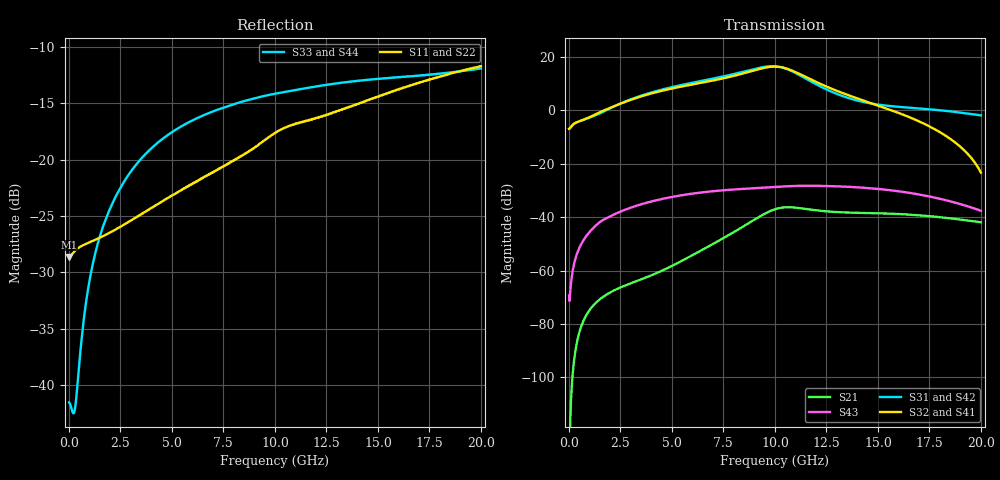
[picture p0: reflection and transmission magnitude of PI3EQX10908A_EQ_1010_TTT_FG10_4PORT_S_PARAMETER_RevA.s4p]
! NPort=4 DATA=2000 NOISE=0 GROUPDELAY=0 COMPLEX_DATAFORMAT=POLAR
! NumOfBlock=1 NumOfParam=0
! .MODEL Smodel S TSTONEFILE=PI3EQX10908A_EQ_1010_TTT_FG10_4PORT_S_PARAMETER_RevA.s4p TYPE=S
!  -- The above .MODEL line can be used for the S element in the netlist.
! The s parameter is extracted from the linear redriver, it is not bi-directional; only s(4,1)s(4,2) and s(3,1)s(3,2)
! should be the insertion loss
!Port definition:
!Port1 = input+
!Port2 = input-
!Port3 = output+
!Port4 = output-
# Hz S MA R  50
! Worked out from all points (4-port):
!   2000 points, 10 MHz to 20 GHz, reference 50 ohm
!   strongest paths, dB at 10 MHz, 5.01 GHz, 10.01 GHz, 15.01 GHz, 20 GHz:
!     S32: -6.9, 8.2, 16.3, 1.8, -23.3
!     S41: -6.9, 8.2, 16.3, 1.8, -23.3
!     S31: -6.9, 8.7, 16.5, 2.1, -1.9
!     S42: -6.9, 8.7, 16.5, 2.1, -1.9
!     S43: -69.4, -32.4, -28.7, -29.5, -37.6
!     S21: -127.2, -58.2, -37.0, -38.6, -41.9
!   lowest |S11| = -28.6 dB at 10 MHz (marker M1), VSWR 1.08, Z = 46.4 - j0.024 ohm
!   |S11| at or under -10 dB: start of sweep to end of sweep
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1e7  0.03701 -179.6  4.341e-07 14.5  0 0.0  0 0.0
     4.341e-07 14.5  0.03701 -179.6  0 0.0  0 0.0
     0.4507 1.1  0.4507 -178.9  0.008374 26.0  0.00034 -27.1
     0.4507 -178.9  0.4507 1.1  0.00034 -27.1  0.008374 26.0
6.85e9  0.08649 -119.6  0.002926 133.9  4.484e-07 62.9  2.294e-07 136.3
        0.002926 134.0  0.08652 -119.6  2.294e-07 136.3  4.484e-07 62.8
        3.821 -51.5  3.517 122.0  0.1617 10.9  0.03013 15.2
        3.518 122.0  3.821 -51.5  0.03013 15.2  0.1617 10.9
9.18e9  0.116 -111.6  0.009814 111.4  2.651e-06 18.1  1.658e-06 115.9
        0.009818 111.4  0.116 -111.6  1.659e-06 115.9  2.651e-06 18.1
        6.164 -111.5  5.847 63.0  0.1889 -7.1  0.035 -8.7
        5.847 63.0  6.165 -111.5  0.035 -8.7  0.1889 -7.1
1.035e10  0.1369 -112.0  0.01505 73.8  4.316e-06 -16.1  4.594e-06 81.4
          0.01506 73.8  0.137 -112.0  4.596e-06 81.5  4.316e-06 -16.2
          6.34 -163.9  6.344 9.6  0.1987 -14.9  0.03735 -20.6
          6.344 9.6  6.341 -163.9  0.03735 -20.6  0.1987 -14.9
1.143e10  0.1478 -113.4  0.01434 42.4  5.025e-06 -26.0  7.712e-06 44.7
          0.01434 42.4  0.1479 -113.4  7.715e-06 44.7  5.024e-06 -26.1
          4.059 155.2  4.338 -34.8  0.207 -21.1  0.03852 -33.7
          4.337 -34.7  4.059 155.2  0.03852 -33.7  0.207 -21.1
1.361e10  0.1718 -111.8  0.01214 14.6  1.366e-05 -36.4  1.654e-05 -5.1
          0.01213 14.7  0.1719 -111.8  1.655e-05 -5.1  1.365e-05 -36.5
          1.679 125.7  1.89 -82.4  0.2216 -32.5  0.03681 -60.1
          1.889 -82.4  1.679 125.7  0.03681 -60.1  0.2216 -32.5
2e10  0.2599 -114.7  0.008018 -40.2  8.927e-05 -147.8  7.211e-05 -138.7
      0.008014 -39.9  0.2601 -114.7  7.212e-05 -138.7  8.925e-05 -147.9
      0.8025 54.9  0.06822 170.9  0.2539 -52.2  0.01317 -136.6
      0.06869 171.5  0.8033 54.9  0.01317 -136.6  0.2539 -52.2
